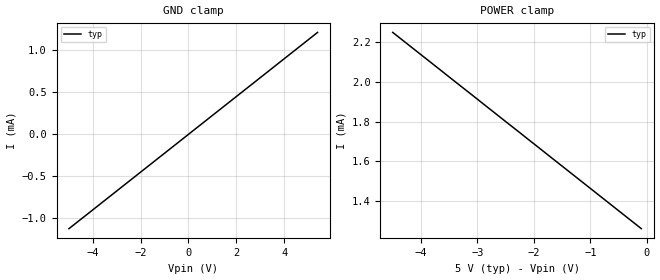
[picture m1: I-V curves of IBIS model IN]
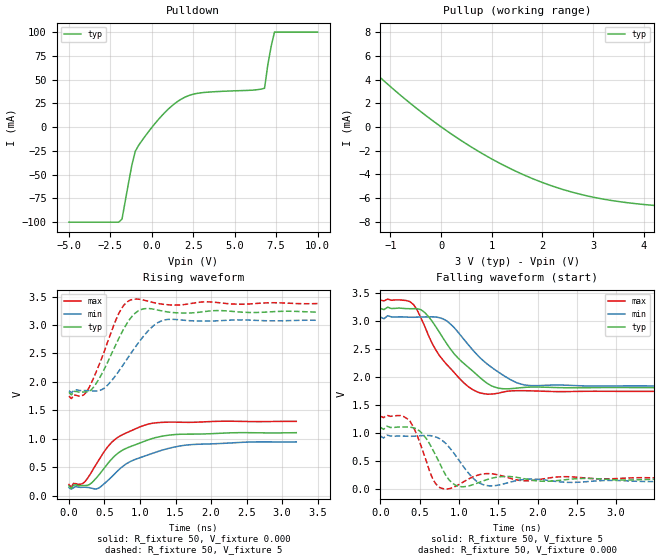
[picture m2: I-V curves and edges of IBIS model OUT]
[IBIS ver]   3.2
[File name]   sample_device_clamp_ref.ibs
[File Rev]   0
[Date]   23/01/2021
[Source]   Company_ABC, data taken from a variety of IBIS files
[Copyright]   None - public sample
|   Component ABC123
[Component]   ABC123
[Manufacturer]   Company_ABC
[Package]
| variable   typ   min   max
R_pkg   46.4m   43.4m   53.1m
L_pkg   2.80nH   1.97nH   2.99nH
C_pkg   0.329pF   0.237pF   0.382pF
[Pin]  signal_name   model_name   R_pin   L_pin   C_pin
1   IN   IN
2   OUT   OUT
3   GND   GND
4   VCC   POWER
| Models and submodels in the file (2): IN (Input), OUT (Output)
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|   Model IN
[Model]   IN
|Signals   R1IN, R2IN
Model_type   Input
Enable   Active-High
Vinl = 0.8V
Vinh = 2.0V
C_comp   0.96pF   0.53pF   1.60pF
[Temperature Range]   25   -40   85
[Voltage Range]   5.00V   4.50V   5.50V
[Pullup Reference]   5.00V   4.50V   5.50V
[Pulldown Reference]   0.00V   -0.5V   0.5V
[POWER Clamp Reference]   5.00V   4.50V   5.50V
[GND Clamp Reference]   0.00V   -0.5V   0.5V
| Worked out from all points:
|   GND clamp passes 1 mA (typ) near -4.44 V on its own axis
[POWER_clamp]
| V(V)  I(typ)   I(min)  I(max)
-4.5V     2.25mA     NA         NA
-2.3V     1.755mA    NA         NA
-1.7V     1.62mA     NA         NA
-100mV    1.26mA     NA         NA
[GND_clamp]
| V(V)  I(typ)   I(min)  I(max)
-5V       -1.127mA   NA         NA
-1V       -226.5uA   NA         NA
5V        1.125mA    NA         NA
5.4V      1.215mA    NA         NA
|   Model OUT
[Model]   OUT
Model_type   Output
Polarity   Non-Inverting
Vmeas = 2.5V
C_comp   0.83pF   0.57pF   1.46pF
[Temperature Range]   25   -40   125
[Voltage Range]   3.00V   2.70V   3.30V
[Pullup Reference]   3.00V   2.70V   3.30V
[Pulldown Reference]   0.00V   -0.5V   0.5V
[POWER Clamp Reference]   3.00V   2.70V   3.30V
[GND Clamp Reference]   0.00V   -0.5V   0.5V
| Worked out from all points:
|   slope of the pulldown table from 0 to 0.45 V, typ, clamps not added: 47.9 ohm
|   slope of the pullup table from 0 to 0.45 V, typ, clamps not added: 345 ohm
|   rising waveform, R_fixture 50, V_fixture 0.000: 20-80 % time 570ps typ, 695ps min, 456ps max; typ from 0.171 V to 1.11 V
|   rising waveform, R_fixture 50, V_fixture 5: 20-80 % time 333ps typ, 427ps min, 300ps max; typ from 1.81 V to 3.23 V
|   falling waveform, R_fixture 50, V_fixture 5: 20-80 % time 501ps typ, 532ps min, 427ps max; typ from 3.23 V to 1.81 V
|   falling waveform, R_fixture 50, V_fixture 0.000: 20-80 % time 216ps typ, 260ps min, 175ps max; typ from 1.1 V to 0.168 V
[Pullup]
| V(V)  I(typ)   I(min)  I(max)
-5V       100mA      NA         NA
-1.8V     10.16mA    NA         NA
-1.6V     5.869mA    NA         NA
-1V       3.425mA    NA         NA
-200mV    653.5uA    NA         NA
1.2V      -3.145mA   NA         NA
2.6V      -5.507mA   NA         NA
3.6V      -6.341mA   NA         NA
5.4V      -6.987mA   NA         NA
5.6V      -7.401mA   NA         NA
5.8V      -15.56mA   NA         NA
10V       -100mA     NA         NA
[Pulldown]
| V(V)  I(typ)   I(min)  I(max)
-5V       -100mA     NA         NA
-2V       -100mA     NA         NA
-1.8V     -96.79mA   NA         NA
-1.2V     -39.62mA   NA         NA
-1V       -25.53mA   NA         NA
0V        -313uA     NA         NA
1V        19.07mA    NA         NA
2.6V      35.07mA    NA         NA
6.8V      40.91mA    NA         NA
7V        65.78mA    NA         NA
7.4V      100mA      NA         NA
10V       100mA      NA         NA
[Ramp]
| variable   typ   min   max
dV/dt_r   90.66V/1uS   47.56V/1uS   145.01V/1uS
dV/dt_f   17.90V/1uS   10.06V/1uS   24.83V/1uS
R_load = 50
[Rising Waveform]
R_fixture   = 50
V_fixture   = 0.000
V_fixture_min   = 0.000
V_fixture_max   = 0.000
|  time   V(typ)   V(min)   V(max)
0s        170.7mV    140.2mV    194.4mV
32ps      123mV      112.3mV    146.7mV
192ps     175.3mV    145.5mV    210mV
288ps     193.3mV    138.8mV    353mV
416ps     355mV      129.3mV    614.8mV
672ps     726.3mV    417.5mV    1.01V
864ps     860.4mV    598.5mV    1.133V
1.12ns    981mV      717.9mV    1.258V
1.696ns   1.08V      893.2mV    1.288V
3.2ns     1.106V     943.9mV    1.305V
[Rising Waveform]
R_fixture   = 50
V_fixture   = 5
V_fixture_min   = 4.5
V_fixture_max   = 5.5
|  time   V(typ)   V(min)   V(max)
0s        1.814V     1.841V     1.747V
210ps     1.821V     1.847V     1.772V
315ps     1.859V     1.841V     1.98V
490ps     2.205V     1.882V     2.511V
700ps     2.76V      2.184V     3.198V
875ps     3.132V     2.506V     3.442V
1.05ns    3.284V     2.803V     3.438V
1.19ns    3.278V     2.987V     3.394V
1.365ns   3.234V     3.092V     3.358V
3.5ns     3.226V     3.082V     3.377V
[Falling Waveform]
R_fixture   = 50
V_fixture   = 5
V_fixture_min   = 4.5
V_fixture_max   = 5.5
|  time   V(typ)   V(min)   V(max)
0s        3.232V     3.079V     3.38V
376ps     3.226V     3.074V     3.354V
517ps     3.208V     3.078V     3.061V
752ps     2.805V     3.065V     2.387V
940ps     2.418V     2.888V     2.084V
1.128ns   2.167V     2.567V     1.822V
1.269ns   1.992V     2.347V     1.718V
1.504ns   1.804V     2.09V      1.715V
1.88ns    1.822V     1.854V     1.757V
4.7ns     1.814V     1.842V     1.747V
[Falling Waveform]
R_fixture   = 50
V_fixture   = 0.000
V_fixture_min   = 0.000
V_fixture_max   = 0.000
|  time   V(typ)   V(min)   V(max)
0s        1.105V     949.6mV    1.304V
378ps     1.107V     942.2mV    1.213V
504ps     1.034V     951.9mV    828.2mV
672ps     691mV      945.9mV    162.8mV
798ps     337.1mV    857.3mV    5.697mV
1.008ns   43.43mV    498.3mV    85.09mV
1.176ns   75.59mV    198.2mV    215.2mV
1.344ns   161.9mV    63.19mV    274mV
1.848ns   178.6mV    172.7mV    145.6mV
4.2ns     167.6mV    140.3mV    196.4mV
